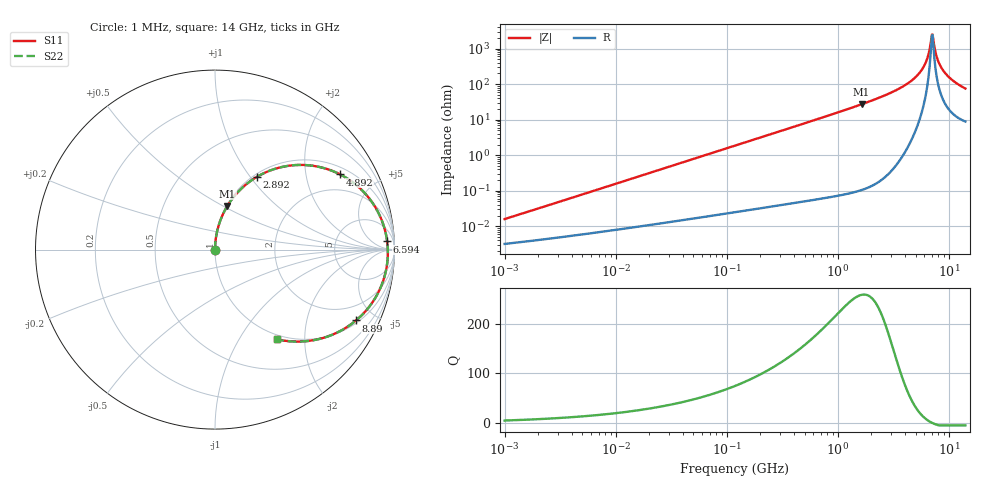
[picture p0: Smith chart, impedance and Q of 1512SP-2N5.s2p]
# MHz  S  MA  R  50
!Freq  MagS11  AngS11  MagS21  AngS21  MagS12  AngS12  MagS22  AngS22
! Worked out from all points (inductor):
!   801 points, 1 MHz to 14 GHz, reference 50 ohm
!   read as one part in series: L = 2.5 nH near 1.049 MHz
!   highest Q = 258 at 1.629 GHz (marker M1), where L = 2.64 nH
!   self-resonance near 7 GHz
!   S11 on the Smith chart (normalised r, x): 1 MHz: 1.00, +0.00; 2.892 GHz: 1.04, +1.08; 4.892 GHz: 1.27, +3.14; 6.594 GHz: 21, +24; 8.89 GHz: 1.13, -3.92; 14 GHz: 0.93, -1.47
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1  0.0001551 78.1  1 -0.0  1 -0.0  0.0001551 78.1
4.958368  0.0007547 85.5  0.9999 -0.0  0.9999 -0.0  0.0007547 85.5
24.29341  0.003688 87.9  0.9999 -0.2  0.9999 -0.2  0.003688 87.9
119.025  0.01806 88.1  0.9996 -1.1  0.9996 -1.1  0.01806 88.1
583.1601  0.08874 84.2  0.9955 -5.4  0.9955 -5.4  0.08873 84.2
1629.484  0.253 74.1  0.9665 -15.6  0.9665 -15.6  0.253 74.1
2857.179  0.4617 60.5  0.8844 -29.2  0.8844 -29.2  0.4616 60.5
2891.522  0.4678 60.0  0.8811 -29.6  0.8811 -29.6  0.4677 60.0
3992.383  0.6657 45.1  0.7375 -44.1  0.7375 -44.1  0.6656 45.1
4891.553  0.8135 31.0  0.5583 -57.3  0.5583 -57.3  0.8134 31.0
5446.89  0.8852 21.7  0.4226 -65.4  0.4226 -65.4  0.8851 21.7
5922.053  0.929 13.7  0.2975 -71.3  0.2975 -71.3  0.9289 13.7
6286.628  0.9504 7.6  0.2003 -73.8  0.2003 -73.8  0.9504 7.6
6594.383  0.9603 2.7  0.1207 -71.5  0.1207 -71.5  0.9603 2.7
6753.864  0.9627 0.2  0.0822 -65.0  0.0822 -65.0  0.9627 0.2
6917.203  0.9634 -2.3  0.04891 -44.7  0.04891 -44.7  0.9634 -2.3
7169.648  0.9611 -6.0  0.04828 31.1  0.04828 31.1  0.9611 -6.0
7888.793  0.9372 -15.6  0.1937 61.0  0.1937 61.0  0.9373 -15.6
8274.98  0.917 -20.2  0.2664 59.4  0.2664 59.4  0.9171 -20.2
8889.995  0.8794 -26.7  0.3664 55.1  0.3664 55.1  0.8795 -26.7
10635.01  0.767 -40.4  0.5609 43.2  0.5609 43.2  0.7674 -40.4
14000  0.607 -55.5  0.7321 28.4  0.7321 28.4  0.6076 -55.5
